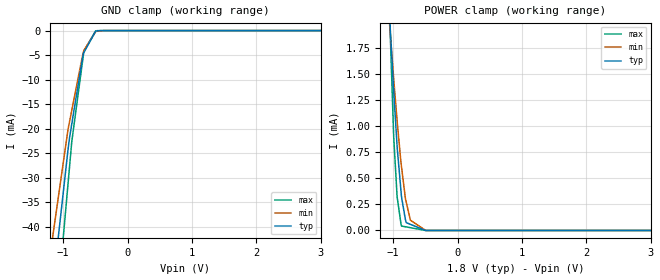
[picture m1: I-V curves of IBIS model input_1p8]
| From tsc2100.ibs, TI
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|   input_1p8 Model
[Model]   input_1p8
Model_type   Input
Vinl = 0.54
Vinh = 1.26
|   typ   min   max
|   (nom PVT)   (fast PVT)   (slow PVT)
|C_comp from frequency sweep method (F=50MHz)
|Average
|C_comp   1.324e-12   1.322e-12   1.330e-12
|C_comp from LC tank measurement(L=1nH)
|Average
|Resonant Frequency(Hz)   4.930e+09   4.940e+09   4.928e+09
C_comp   1.043e-12   1.039e-12   1.044e-12
| Where nom  PVT is Nominal Process, 1.8V, 26C
|   Fast PVT is Strong Process,  1.98V, -40C
|   Slow PVT is Weak Process,   1.62V, 86C
[Model Spec]
|Subparameter   typ   min   max
Vinh   1.26   1.134   1.386
Vinl   0.54   0.486   0.594
[Voltage Range]   1.8   1.62   1.98
|Ambient Temperature   25   85   -40
|Junction Temperature
[Temperature Range]   26   86   -40
[Power Clamp Reference]   1.8   1.62   1.98
[GND Clamp Reference]   0   0   0
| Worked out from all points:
|   GND clamp passes 1 mA (typ) near -0.53 V on its own axis
|   POWER clamp passes 1 mA (typ) near -0.96 V on its own axis
[GND Clamp]
|   Voltage   I(typ)   I(min)   I(max)
-1.8V     -243.8mA   -115.3mA   -355.4mA
-1.176V   -53.94mA   -43.24mA   -68.31mA
-925mV    -24.33mA   -20.2mA    -31.32mA
-900mV    -21.75mA   -18.51mA   -27.63mA
-865.3mV  -18.96mA   -16.19mA   -22.56mA
-693.4mV  -5.165mA   -4.748mA   -5.738mA
-687.6mV  -4.702mA   -4.491mA   -5.174mA
-677.2mV  -4.454mA   -4.027mA   -4.153mA
-495mV    -128.5uA   -227.4uA   -54.51uA
-315.9mV  -1.005uA   -2.528uA   -73.24nA
3.6V      0A         0A         0A
[POWER Clamp]
|   Voltage   I(typ)   I(min)   I(max)
-1.8V     11.73mA    8.527mA    19.35mA
-1.085V   2.421mA    2.215mA    2.616mA
-1.046V   1.94mA     1.895mA    1.894mA
-992mV    1.34mA     1.456mA    910.2uA
-938.5mV  808.3uA    1.052mA    323.2uA
-882.9mV  409.2uA    677.3uA    82.81uA
-871.2mV  326.3uA    615uA      42.39uA
-810mV    104.7uA    307.5uA    35.49uA
-795.6mV  74.49uA    268.7uA    33.87uA
-732.2mV  58.79uA    98.08uA    26.73uA
-494.1mV  0A         161.5nA    0A
3.6V      0A         0A         0A
